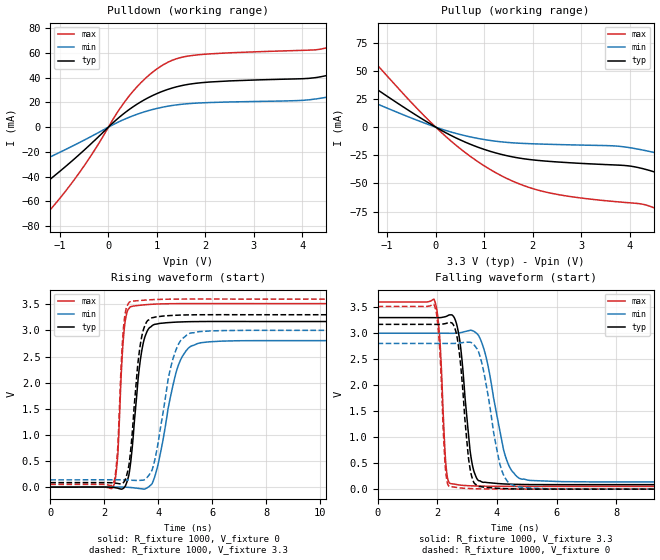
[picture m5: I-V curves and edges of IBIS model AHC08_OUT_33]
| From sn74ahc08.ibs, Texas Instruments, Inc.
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[Model]   AHC08_OUT_33
Model_type  Output
Vref =   0
Rref =   1000
Cref =   50p
Vmeas =   1.65
| variable   typ   min   max
C_comp   3.07pF   2.15pF   3.99pF
| C_pullup   3.13pF   2.15pF   3.99pF
| C_pulldown   3.01pF   2.25pF   3.81pF
[Temperature Range]   40   100   -40
| Ambient temperature   25   85   -40
[Voltage range]   3.3   3   3.6
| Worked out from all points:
|   slope of the pulldown table from 0 to 0.495 V, typ, clamps not added: 30.7 ohm
|   slope of the pullup table from 0 to 0.495 V, typ, clamps not added: 44.5 ohm
|   rising waveform, R_fixture 1000, V_fixture 0: 20-80 % time 354ps typ, 642ps min, 193ps max; typ from 0 V to 3.17 V
|   falling waveform, R_fixture 1000, V_fixture 3.3: 20-80 % time 305ps typ, 563ps min, 170ps max; typ from 3.3 V to 0.086 V
|   rising waveform, R_fixture 1000, V_fixture 3.3: 20-80 % time 332ps typ, 584ps min, 188ps max; typ from 0.086 V to 3.3 V
|   falling waveform, R_fixture 1000, V_fixture 0: 20-80 % time 283ps typ, 506ps min, 171ps max; typ from 3.17 V to 0 V
[Pulldown]
| AHC08_OUT_33
|   Voltage   I(typ)   I(min)   I(max)
-5.5V     -152.9mA   -94.93mA   -192.9mA
-4.71V    -134.2mA   -82.55mA   -171.9mA
-2.665V   -84.6mA    -49.69mA   -117.9mA
-1.525V   -52.13mA   -29.98mA   -80.77mA
-650mV    -23.85mA   -13.49mA   -39.52mA
510mV     16.49mA    9.234mA    29.1mA
1.48V     33.3mA     18.35mA    56.14mA
4.47V     41.42mA    23.96mA    63.83mA
5.395V    53.43mA    32.73mA    81.21mA
6.825V    82.47mA    52.85mA    124.5mA
8.56V     127.4mA    82.81mA    191.5mA
11V       203.2mA    129.3mA    308.7mA
[Pullup]
| AHC08_OUT_33
|   Voltage   I(typ)   I(min)   I(max)
-5.5V     176.9mA    104.5mA    308.5mA
-4.615V   144.4mA    86.84mA    247.4mA
-2.955V   87.61mA    53.95mA    146.3mA
-1.865V   53.12mA    32.88mA    87.96mA
405mV     -9.291mA   -5.409mA   -15.58mA
1.305V    -23.67mA   -12.82mA   -42.01mA
2.17V     -29.79mA   -15.03mA   -56.61mA
4.33V     -37.5mA    -20.85mA   -69.06mA
5.33V     -52.54mA   -31.43mA   -89.21mA
7.29V     -90.96mA   -57.06mA   -136.9mA
9.55V     -140.3mA   -89.73mA   -194.5mA
11V       -173.5mA   -111.7mA   -232.6mA
[Ramp]
| AHC08_OUT_33
| variable   typ   min   max
dV/dt_r   1.93/3.86E-10   1.71/6.74E-10   2.13/2.01E-10
dV/dt_f   1.96/3.20E-10   1.75/5.90E-10   2.16/1.77E-10
R_load = 1000
[Rising Waveform]
| AHC08_OUT_33
R_fixture =   1000
C_fixture =   0
L_fixture =   0
V_fixture =   0
V_fixture_min = 0
V_fixture_max = 0
|   Time   V(typ)   V(min)   V(max)
0s        168.2pV    387.5pV    67.12pV
2.345ns   -6.404mV   775uV      21.76mV
2.5ns     -20.42mV   1.01mV     590.2mV
2.75ns    -4.398mV   -736.1uV   3.064V
3.085ns   1.035V     -13.1mV    3.469V
3.345ns   2.454V     -29.47mV   3.483V
3.625ns   3.018V     -3.217mV   3.497V
4.76ns    3.162V     2.349V     3.514V
5.59ns    3.171V     2.765V     3.515V
50ns      3.17V      2.803V     3.514V
[Falling Waveform]
| AHC08_OUT_33
R_fixture =   1000
C_fixture =   0
L_fixture =   0
V_fixture =   3.3
V_fixture_min = 3
V_fixture_max = 3.6
|   Time   V(typ)   V(min)   V(max)
0s        3.3V       3V         3.6V
1.905ns   3.299V     3V         3.636V
2.09ns    3.299V     3V         2.873V
2.33ns    3.331V     2.999V     268.3mV
2.775ns   2.78V      3.01V      77.62mV
3.1ns     749.6mV    3.054V     63.72mV
3.32ns    212.7mV    2.998V     59.47mV
4.335ns   97mV       548.4mV    52.6mV
5.105ns   87.26mV    166.5mV    51.83mV
50ns      86.09mV    139.4mV    52.22mV
[Rising Waveform]
| AHC08_OUT_33
R_fixture =   1000
C_fixture =   0
L_fixture =   0
V_fixture =   3.3
V_fixture_min = 3
V_fixture_max = 3.6
|   Time   V(typ)   V(min)   V(max)
0s        86.09mV    139.4mV    52.22mV
2.34ns    80.76mV    139.7mV    79.42mV
2.5ns     70.45mV    139.7mV    745.4mV
2.735ns   101.3mV    137.8mV    3.162V
3.055ns   1.143V     130.7mV    3.562V
3.3ns     2.591V     129mV      3.572V
3.565ns   3.158V     171.9mV    3.583V
4.625ns   3.291V     2.579V     3.6V
5.515ns   3.301V     2.978V     3.601V
50ns      3.3V       3V         3.6V
[Falling Waveform]
| AHC08_OUT_33
R_fixture =   1000
C_fixture =   0
L_fixture =   0
V_fixture =   0
V_fixture_min = 0
V_fixture_max = 0
|   Time   V(typ)   V(min)   V(max)
0s        3.17V      2.803V     3.514V
1.905ns   3.17V      2.803V     3.537V
2.08ns    3.17V      2.802V     2.735V
2.275ns   3.185V     2.802V     402.7mV
2.42ns    3.208V     2.802V     45.99mV
3.105ns   379mV      2.826V     10.39mV
3.4ns     48.56mV    2.62V      5.542mV
4.165ns   11.32mV    358.9mV    865.7uV
4.93ns    1.708mV    29.91mV    -226.3uV
50ns      8.456nV    -14.24nV   -24.23pV
